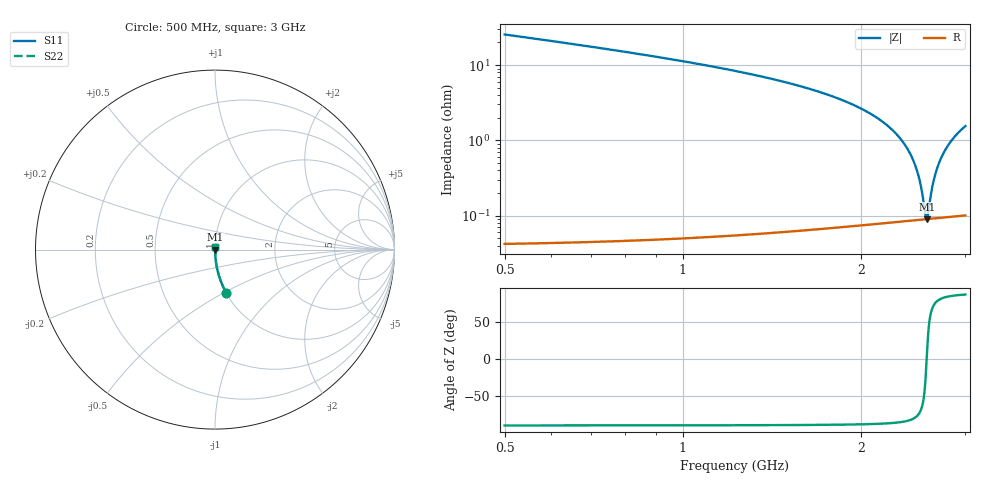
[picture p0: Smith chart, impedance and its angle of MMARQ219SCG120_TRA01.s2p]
! MMARQ219SCG120_TRA01  S-PARAMETER MODEL  ( General Type )
! Model Generated by TAIYO YUDEN Corporation (http://www.ty-top.com)
! Version 1.0
! TAIYO YUDEN Control No. 180601
! Copyright(c) 2018 TAIYO YUDEN CO.,LTD. All Rights Reserved.
! Product Description (link to TY-COMPAS)
! https://ds.yuden.co.jp/TYCOMPAS/or/detail?pn=MMARQ219SCG120JTRA01&u=M
! Products Name : Multilayer Ceramic Capacitors
! Characteristics :
!  Capacitance : 12 pF , Rated Voltage : 250V , TCC : CG / C0G
!  Case Size : 2.0 x 1.25 / 0.079 x 0.049 [mm/inch] , Thickness : 0.85 / 0.033 [mm/inch]
!  (Conditions: Temperature = 25 degC , DC Bias Current/Voltage = 0A / 0V)
! External Node Assignments :
!  1  o---| |---o  2
! GND o---------o GND
! Frequency Range : 500MHz  -  3000MHz  [ 401 STEP ]
# MHz S RI R 50
! Freq[MHz].  S11 Real  S11 Imag  S21 Real  S21 Imag  S12 Real  S12 Imag  S22 Real  S22 Imag
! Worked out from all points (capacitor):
!   401 points, 500 MHz to 3 GHz, reference 50 ohm
!   read as one part in series: C = 12 pF near 512.5 MHz
!   lowest |Z| = 89.7 mohm at 2.581 GHz (marker M1)
!   series resonance near 2.581 GHz, so ESL is about 320 pH
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500  0.0615 -0.2395  0.9385 0.2395  0.9385 0.2395  0.0615 -0.2395
918.75  0.0161 -0.1239  0.9839 0.1239  0.9839 0.1239  0.0161 -0.1239
1337.5  0.00578 -0.072  0.9942 0.072  0.9942 0.072  0.00578 -0.072
1750  0.00233 -0.0407  0.9977 0.0407  0.9977 0.0407  0.00233 -0.0407
1987.5  0.00147 -0.027  0.9985 0.027  0.9985 0.027  0.00147 -0.027
2168.75  0.0011 -0.0179  0.9989 0.0179  0.9989 0.0179  0.0011 -0.0179
2325  0.000942 -0.0107  0.9991 0.0107  0.9991 0.0107  0.000942 -0.0107
2387.5  0.000908 -0.00796  0.9991 0.00796  0.9991 0.00796  0.000908 -0.00796
2437.5  0.000892 -0.00584  0.9991 0.00584  0.9991 0.00584  0.000892 -0.00584
2475  0.000886 -0.00428  0.9991 0.00428  0.9991 0.00428  0.000886 -0.00428
2506.25  0.000885 -0.003  0.9991 0.003  0.9991 0.003  0.000885 -0.003
2531.25  0.000887 -0.00198  0.9991 0.00198  0.9991 0.00198  0.000887 -0.00198
2568.75  0.000893 -0.000479  0.9991 0.000479  0.9991 0.000479  0.000893 -0.000479
2581.25  0.000896 1.69e-05  0.9991 -1.69e-05  0.9991 -1.69e-05  0.000896 1.69e-05
2587.5  0.000898 0.000264  0.9991 -0.000264  0.9991 -0.000264  0.000898 0.000264
2631.25  0.000913 0.00198  0.9991 -0.00198  0.9991 -0.00198  0.000913 0.00198
2650  0.000921 0.0027  0.9991 -0.0027  0.9991 -0.0027  0.000921 0.0027
2681.25  0.000937 0.0039  0.9991 -0.0039  0.9991 -0.0039  0.000937 0.0039
2725  0.000965 0.00555  0.999 -0.00555  0.999 -0.00555  0.000965 0.00555
2781.25  0.00101 0.00764  0.999 -0.00764  0.999 -0.00764  0.00101 0.00764
2843.75  0.00106 0.00992  0.9989 -0.00992  0.9989 -0.00992  0.00106 0.00992
3000  0.00124 0.0154  0.9988 -0.0154  0.9988 -0.0154  0.00124 0.0154
